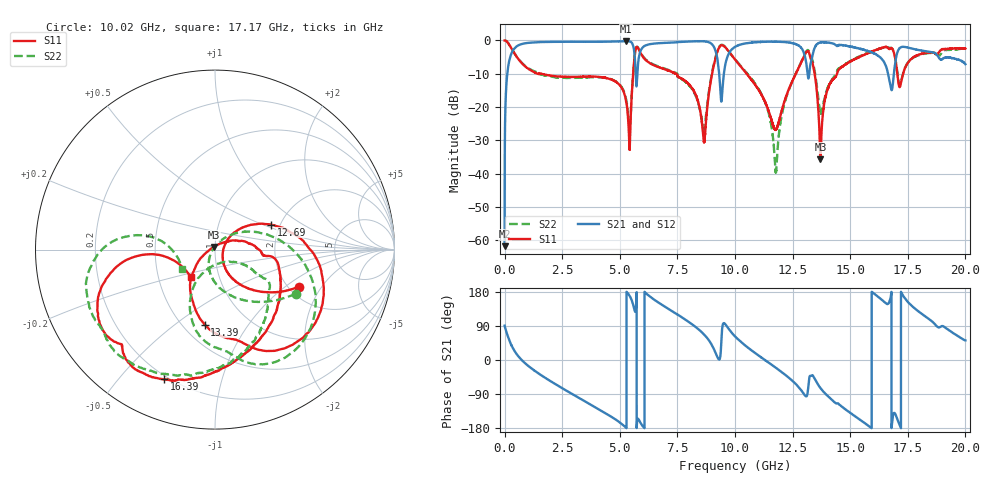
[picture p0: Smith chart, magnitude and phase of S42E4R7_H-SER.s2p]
! Created Wed Nov 25 21:46:29 2020
# khz S ma R 50
! 2 Port Network Data from SP1.SP block
! freq  magS11  angS11  magS21  angS21  magS12  angS12  magS22  angS22
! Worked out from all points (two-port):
!   20001 points, 300 kHz to 20 GHz, reference 50 ohm
!   highest |S21| = -0.21 dB at 5.27 GHz (marker M1); lowest = -61.8 dB at 300 kHz (marker M2)
!   |S21| within 3 dB of the highest: 343 MHz to 5.624 GHz (5.281 GHz wide, 177 % of centre); 5.895 GHz to 9.158 GHz (3.263 GHz wide, 43.4 % of centre)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
!   lowest |S11| = -35.8 dB at 13.71 GHz (marker M3), VSWR 1.03, Z = 49.4 + j1.5 ohm
!   |S11| at or under -10 dB: 1.594 GHz to 5.577 GHz (3.983 GHz wide, 111 % of centre); 7.436 GHz to 9.005 GHz (1.569 GHz wide, 19.1 % of centre); 10.51 GHz to 12.64 GHz (2.132 GHz wide, 18.4 % of centre)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
!   |S22| runs from -39.7 to 0.0 dB; largest |S21 - S12| = 0.019
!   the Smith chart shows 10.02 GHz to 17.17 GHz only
!   S11 on the Smith chart (normalised r, x): 10.02 GHz: 2.26, -1.26; 12.69 GHz: 1.80, +0.57; 13.39 GHz: 0.64, -0.65; 16.39 GHz: 0.18, -0.67; 17.17 GHz: 0.73, -0.24
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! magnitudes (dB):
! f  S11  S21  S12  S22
! 300 kHz  0.0  -61.8  -61.8  0.0
! 117.3 MHz  -0.5  -9.9  -9.9  -0.5
! 361.3 MHz  -3.1  -3.0  -3.0  -3.1
! 3.334 GHz  -10.9  -0.4  -0.4  -11.2
! 5.27 GHz  -18.0  -0.2  -0.2  -17.6
! 5.434 GHz  -32.2  -0.3  -0.3  -28.3
! 5.748 GHz  -1.9  -11.5  -11.5  -1.9
! 6.667 GHz  -8.0  -0.8  -0.9  -7.8
! 8.648 GHz  -30.4  -0.3  -0.3  -27.1
! 9.269 GHz  -2.7  -7.1  -7.2  -2.5
! 10 GHz  -5.7  -1.9  -1.9  -5.6
! 10.02 GHz  -5.8  -1.9  -1.9  -5.8
! 11.77 GHz  -26.9  -0.4  -0.4  -39.4
! 12.69 GHz  -9.3  -1.2  -1.2  -9.2
! 13.33 GHz  -6.2  -5.5  -5.5  -5.4
! 13.39 GHz  -7.5  -3.6  -3.7  -6.7
! 13.71 GHz  -35.8  -0.6  -0.6  -21.7
! 14.53 GHz  -8.6  -1.4  -1.3  -8.3
! 16.39 GHz  -2.2  -5.7  -5.8  -2.3
! 16.67 GHz  -2.4  -10.8  -11.0  -2.3
! 17.17 GHz  -13.7  -2.1  -2.2  -13.4
! 20 GHz  -2.5  -7.1  -7.1  -2.3
